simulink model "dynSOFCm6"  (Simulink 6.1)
settings: Solver=ode15s  StartTime=0.0  StopTime=1000  FixedStep=0.001  MinStep=1e-10  RelTol=1e-3
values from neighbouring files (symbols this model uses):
  A = 1e-4    (= 0.0001)    [dynSOFC_par.m]
  Aa = r3^2*(4-pi)    (= 0.000103867288916)    [dynSOFC_par.m]
  Ac = pi*(r2^2-r1^2)    (= 0.000122508290482)    [dynSOFC_par.m]
  At = pi*r0^2    (= 7.85398163397e-05)    [dynSOFC_par.m]
  C = 300e-6    (= 0.0003)    [dynSOFC_par.m]
  Cpc = 740    [dynSOFC_par.m]
  Cpt = 1217.7    [dynSOFC_par.m]
  D_a = 0.273*2*r3    (= 0.006006)    [dynSOFC_par.m]
  D_c = 2*(r2-r1)    (= 0.00532)    [dynSOFC_par.m]
  delta = 5.67e-8    (= 5.67e-08)    [dynSOFC_par.m]
  dVa = Aa*A/(2*pi*r3)    (= 1.50281749604e-07)    [dynSOFC_par.m]
  dVc = Ac*A/(2*pi*r3)    (= 1.77252727273e-07)    [dynSOFC_par.m]
  dVt = At*A/(2*pi*r3)    (= 1.13636363636e-07)    [dynSOFC_par.m]
  Ea = 1.1e5    (= 110000)    [dynSOFC_par.m]
  Ec = 1.2e5    (= 120000)    [dynSOFC_par.m]
  Ems1 = 0.4    [dynSOFC_par.m]
  Ems2 = 0.9    [dynSOFC_par.m]
  F = 96487    [dynSOFC_par.m]
  F21 = 0.69    [dynSOFC_par.m]
  K = 10    [dynSOFC_par.m]
  La = 0.1e-3    (= 0.0001)    [dynSOFC_par.m]
  Lc = 2.21e-3    (= 0.00221)    [dynSOFC_par.m]
  Le = 0.04e-3    (= 4e-05)    [dynSOFC_par.m]
  R = 8.314/101325    (= 8.20528003948e-05)    [dynSOFC_par.m]
  r0 = 5e-3    (= 0.005)    [dynSOFC_par.m]
  r1 = 6e-3    (= 0.006)    [dynSOFC_par.m]
  r2 = 8.66e-3    (= 0.00866)    [dynSOFC_par.m]
  r3 = 11e-3    (= 0.011)    [dynSOFC_par.m]
  Ro = 0.01    [dynSOFC_par.m]
  Rouc = 4592    [dynSOFC_par.m]
  Rout = 3900    [dynSOFC_par.m]
  x_ini = [    [dynSOFC_par.m]
libraries: simulink x25
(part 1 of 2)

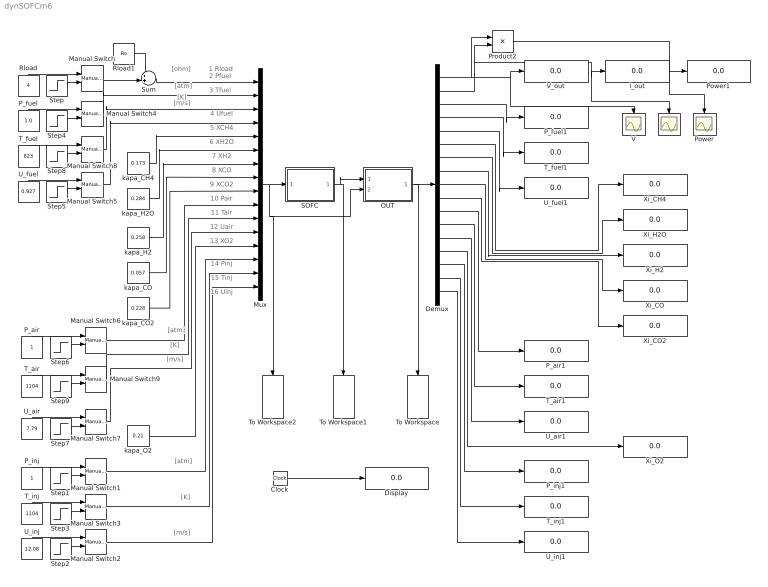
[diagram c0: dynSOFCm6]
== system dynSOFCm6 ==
  note: [ohm]
  note: [m/s]
  note: [atm]
  note: 1 Rload
  note: 3 Tfuel
  note: 5 XCH4
  note: [K]
  note: 6 XH2O
  note: 7 XH2
  note: 8 XCO
  note: 9 XCO2
  note: 4 Ufuel
  note: 2 Pfuel
  note: 10 Pair
  note: 11 Tair
  note: 12 Uair
  note: 13 XO2
  note: 14 Pinj
  note: 15 Tinj
  note: 16 Uinj
  note: [m/s]
  note: [atm]
  note: [K]
  note: [m/s]
  note: [atm]
  note: [K]
  Clock : Clock
  Demux : Demux  Outputs=17
  Display : Display
  I : Scope
  I_out : Display
  Manual Switch{,1..9} (10 alike) : simulink/Signal Routing/Manual Switch  sw=1  action=0
  Mux : Mux  Inputs=16
  OUT : Subsystem
  P_air : Constant  Orientation=up
  P_air1 : Display
  P_fuel : Constant  Orientation=up  Value=1.0
  P_fuel1 : Display
  P_inj : Constant  Orientation=up
  P_inj1 : Display
  Power : Scope
  Power1 : Display
  Product2 : Product
  Rload : Constant  Orientation=up  Value=4
  Rload1 : Constant  Value=Ro
  SOFC : Subsystem
  Step : Step  Time=100  Before=4  After=2
  Step1 : Step  Time=0.05  Before=0.03  After=0.03*0.5
  Step2 : Step  Time=0.05  Before=0.03  After=0.03*0.5
  Step3 : Step  Time=0.05  Before=0.03  After=0.03*0.5
  Step4 : Step  Time=100  Before=1  After=1.05
  Step5 : Step  Time=100  Before=0.927
  Step6 : Step  Time=100  Before=1  After=1.05
  Step7 : Step  Time=100  Before=7.79  After=8
  Step8 : Step  Time=100  Before=823  After=873
  Step9 : Step  Time=100  Before=1104  After=1154
  Sum : Sum  Inputs=++|
  T_air : Constant  Orientation=up  Value=1104
  T_air1 : Display
  T_fuel : Constant  Orientation=up  Value=823
  T_fuel1 : Display
  T_inj : Constant  Orientation=up  Value=1104
  T_inj1 : Display
  To Workspace : ToWorkspace  VariableName=y  SaveFormat=Array
  To Workspace1 : ToWorkspace  VariableName=x  SaveFormat=Array
  To Workspace2 : ToWorkspace  VariableName=u  SaveFormat=Array
  U_air : Constant  Orientation=up  Value=7.79
  U_air1 : Display
  U_fuel : Constant  Orientation=up  Value=0.927
  U_fuel1 : Display
  U_inj : Constant  Orientation=up  Value=12.08
  U_inj1 : Display
  V : Scope
  V_out : Display
  Xi_CH4 : Display
  Xi_CO : Display
  Xi_CO2 : Display
  Xi_H2 : Display
  Xi_H2O : Display
  Xi_O2 : Display
  kapa_CH4 : Constant  Value=0.173
  kapa_CO : Constant  Value=0.057
  kapa_CO2 : Constant  Value=0.228
  kapa_H2 : Constant  Value=0.258
  kapa_H2O : Constant  Value=0.284
  kapa_O2 : Constant  Value=0.21
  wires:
  Mux/1 -> SOFC/1(u), OUT/2(u), To Workspace2/1
  SOFC/1(x) -> OUT/1(x), To Workspace1/1
  OUT/1(y) -> Demux/1, To Workspace/1
  Demux/1 -> Product2/1, V_out/1, V/1
  Demux/2 -> Product2/2, I_out/1, I/1
  Rload/1 -> Manual Switch/1
  Step/1 -> Manual Switch/2
  Clock/1 -> Display/1
  Sum/1 -> Mux/1
  P_fuel/1 -> Manual Switch4/1
  Step4/1 -> Manual Switch4/2
  U_fuel/1 -> Manual Switch5/1
  Step5/1 -> Manual Switch5/2
  P_air/1 -> Manual Switch6/1
  Step6/1 -> Manual Switch6/2
  U_air/1 -> Manual Switch7/1
  Step7/1 -> Manual Switch7/2
  T_fuel/1 -> Manual Switch8/1
  Step8/1 -> Manual Switch8/2
  T_air/1 -> Manual Switch9/1
  Step9/1 -> Manual Switch9/2
  Manual Switch5/1 -> Mux/4
  Manual Switch4/1 -> Mux/2
  Manual Switch/1 -> Sum/2
  Rload1/1 -> Sum/1
  Manual Switch8/1 -> Mux/3
  P_inj/1 -> Manual Switch1/1
  U_inj/1 -> Manual Switch2/1
  Step2/1 -> Manual Switch2/2
  T_inj/1 -> Manual Switch3/1
  Step3/1 -> Manual Switch3/2
  kapa_CH4/1 -> Mux/5
  kapa_H2O/1 -> Mux/6
  kapa_H2/1 -> Mux/7
  kapa_CO/1 -> Mux/8
  kapa_CO2/1 -> Mux/9
  Manual Switch6/1 -> Mux/10
  Manual Switch9/1 -> Mux/11
  Manual Switch7/1 -> Mux/12
  kapa_O2/1 -> Mux/13
  Manual Switch1/1 -> Mux/14
  Manual Switch3/1 -> Mux/15
  Manual Switch2/1 -> Mux/16
  Product2/1 -> Power1/1, Power/1
  Demux/3 -> P_fuel1/1
  Demux/4 -> T_fuel1/1
  Demux/5 -> U_fuel1/1
  Demux/6 -> Xi_CH4/1
  Demux/7 -> Xi_H2O/1
  Demux/8 -> Xi_H2/1
  Demux/9 -> Xi_CO/1
  Demux/10 -> Xi_CO2/1
  Demux/11 -> P_air1/1
  Demux/12 -> T_air1/1
  Demux/13 -> U_air1/1
  Demux/14 -> Xi_O2/1
  Demux/15 -> P_inj1/1
  Demux/16 -> T_inj1/1
  Demux/17 -> U_inj1/1
  Step1/1 -> Manual Switch1/2

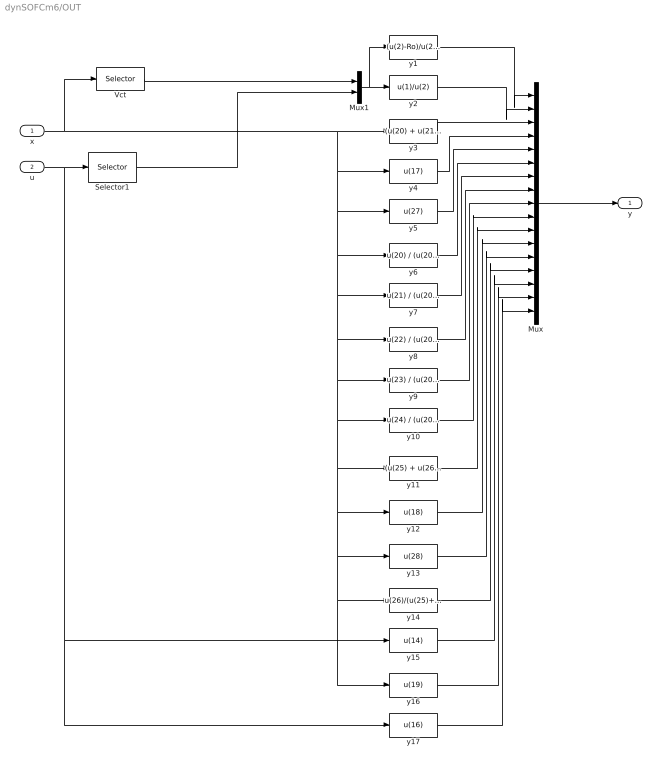
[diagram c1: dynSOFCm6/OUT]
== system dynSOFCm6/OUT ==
  x : Inport  Port=1  LatchInput=off
  u : Inport  Port=2  LatchInput=off
  Mux : Mux  Inputs=17
  Mux1 : Mux  Inputs=2
  Selector1 : Selector  Elements=[1]  InputPortWidth=16
  Vct : Selector  Elements=[1]  InputPortWidth=28
  y1 : Fcn  Expr=(u(2)-Ro)/u(2)*u(1)
  y10 : Fcn  Expr=u(24) / (u(20) + u(21) + u(22) + u(23) + u(24))
  y11 : Fcn  Expr=(u(25) + u(26)) * R * u(18) / dVc
  y12 : Fcn  Expr=u(18)
  y13 : Fcn  Expr=u(28)
  y14 : Fcn  Expr=u(26)/(u(25)+u(26))
  y15 : Fcn  Expr=u(14)
  y16 : Fcn  Expr=u(19)
  y17 : Fcn  Expr=u(16)
  y2 : Fcn  Expr=u(1)/u(2)
  y3 : Fcn  Expr=(u(20) + u(21) + u(22) + u(23) + u(24)) * R * u(17) /dVa
  y4 : Fcn  Expr=u(17)
  y5 : Fcn  Expr=u(27)
  y6 : Fcn  Expr=u(20) / (u(20) + u(21) + u(22) + u(23) + u(24))
  y7 : Fcn  Expr=u(21) / (u(20) + u(21) + u(22) + u(23) + u(24))
  y8 : Fcn  Expr=u(22) / (u(20) + u(21) + u(22) + u(23) + u(24))
  y9 : Fcn  Expr=u(23) / (u(20) + u(21) + u(22) + u(23) + u(24))
  y : Outport
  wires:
  x/1 -> Vct/1, y3/1, y4/1, y5/1, y6/1, y7/1, y8/1, y9/1, y10/1, y12/1, y13/1, y16/1, y14/1, y11/1
  u/1 -> Selector1/1, y15/1, y17/1
  y2/1 -> Mux/2
  Mux/1 -> y/1
  Selector1/1 -> Mux1/2
  Mux1/1 -> y2/1, y1/1
  y1/1 -> Mux/1
  Vct/1 -> Mux1/1
  y3/1 -> Mux/3
  y4/1 -> Mux/4
  y5/1 -> Mux/5
  y6/1 -> Mux/6
  y7/1 -> Mux/7
  y8/1 -> Mux/8
  y9/1 -> Mux/9
  y10/1 -> Mux/10
  y11/1 -> Mux/11
  y12/1 -> Mux/12
  y13/1 -> Mux/13
  y14/1 -> Mux/14
  y15/1 -> Mux/15
  y16/1 -> Mux/16
  y17/1 -> Mux/17

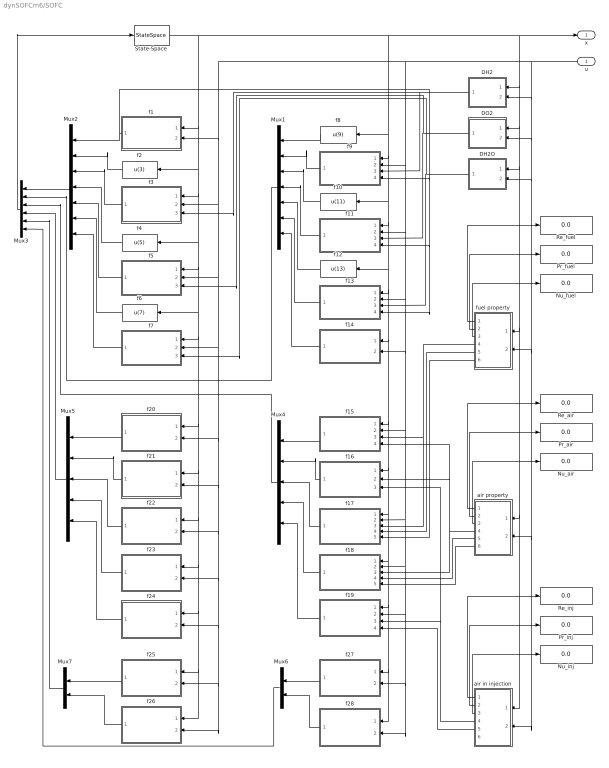
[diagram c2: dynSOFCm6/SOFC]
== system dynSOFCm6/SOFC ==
  u : Inport  Orientation=left  Port=1  LatchInput=off
  DH2 : Subsystem  Orientation=left
  DH2O : Subsystem  Orientation=left
  DO2 : Subsystem  Orientation=left
  Mux1 : Mux  Orientation=left  Inputs=7
  Mux2 : Mux  Orientation=left  Inputs=7
  Mux3 : Mux  Orientation=left  Inputs=6
  Mux4 : Mux  Orientation=left  Inputs=5
  Mux5 : Mux  Orientation=left  Inputs=5
  Mux6 : Mux  Orientation=left  Inputs=2
  Mux7 : Mux  Orientation=left  Inputs=2
  Nu_air : Display
  Nu_fuel : Display
  Nu_inj : Display
  Pr_air : Display
  Pr_fuel : Display
  Pr_inj : Display
  Re_air : Display
  Re_fuel : Display
  Re_inj : Display
  State-Space : StateSpace  A=zeros(28,28)  B=eye(28,28)  C=eye(28,28)  D=zeros(28,28)  X0=x_ini
  air in injection : Subsystem  Orientation=left
  air property : Subsystem  Orientation=left
  f1 : Subsystem  Orientation=left
  f10 : Fcn  Orientation=left  Expr=u(11)
  f11 : Subsystem  Orientation=left
  f12 : Fcn  Orientation=left  Expr=u(13)
  f13 : Subsystem  Orientation=left
  f14 : Subsystem  Orientation=left
  f15 : Subsystem  Orientation=left
  f16 : Subsystem  Orientation=left
  f17 : Subsystem  Orientation=left
  f18 : Subsystem  Orientation=left
  f19 : Subsystem  Orientation=left
  f2 : Fcn  Orientation=left  Expr=u(3)
  f20 : Subsystem  Orientation=left
  f21 : Subsystem  Orientation=left
  f22 : Subsystem  Orientation=left
  f23 : Subsystem  Orientation=left
  f24 : Subsystem  Orientation=left
  f25 : Subsystem  Orientation=left
  f26 : Subsystem  Orientation=left
  f27 : Subsystem  Orientation=left
  f28 : Subsystem  Orientation=left
  f3 : Subsystem  Orientation=left
  f4 : Fcn  Orientation=left  Expr=u(5)
  f5 : Subsystem  Orientation=left
  f6 : Fcn  Orientation=left  Expr=u(7)
  f7 : Subsystem  Orientation=left
  f8 : Fcn  Orientation=left  Expr=u(9)
  f9 : Subsystem  Orientation=left
  fuel property : Subsystem  Orientation=left
  x : Outport
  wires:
  State-Space/1 -> f1/1(x), f2/1, f3/1(x), f4/1, f5/1(x), f6/1, f7/1(x), f20/1(x), f21/1(x), f22/1(x), f23/1(x), f24/1(x), f26/1(x), f25/1(x), f8/1, f9/1(x), f10/1, f11/1(x), f13/1(x), f14/1(x), f15/1(x), f16/1(x), f17/1(x), f18/1(x), f19/1(x), f27/1(x), f28/1(x), f12/1, x/1, DH2/1(x), DO2/1(x), DH2O/1(x), fuel property/1(x), air property/1(x), air in injection/1(x)
  f3/1(dot x3) -> Mux2/3
  f2/1 -> Mux2/2
  f1/1(dot x1) -> Mux2/1, f9/4(dotx1), f11/4(dot x1), f13/4(dot x1)
  f4/1 -> Mux2/4
  f5/1(dot x5) -> Mux2/5
  f6/1 -> Mux2/6
  f7/1(dot x7) -> Mux2/7
  f8/1 -> Mux1/1
  f9/1(dot x9) -> Mux1/2
  f10/1 -> Mux1/3
  f11/1(dot x11) -> Mux1/4
  f12/1 -> Mux1/5
  f13/1(dot x13) -> Mux1/6
  f14/1(dot x14) -> Mux1/7
  Mux2/1 -> Mux3/1
  Mux3/1 -> State-Space/1
  u/1 -> f1/2(u), f3/2(u), f5/2(u), f7/2(u), f20/2(u), f21/2(u), f22/2(u), f23/2(u), f24/2(u), f26/2(u), f25/2(u), f9/2(u), f13/2(u), f14/2(u), f15/2(u), f17/2(u), f18/2(u), f19/2(u), f27/2(u), f28/2(u), f11/2(u), DH2/2(u), DO2/2(u), DH2O/2(u), fuel property/2(u), air property/2(u), air in injection/2(u)
  DH2/1(DH2) -> f3/3(DH2), f9/3(DH2)
  DO2/1(DO2) -> f5/3(DO2), f11/3(DO2)
  DH2O/1(DH2O) -> f7/3(DH2O), f13/3(DH2O)
  Mux1/1 -> Mux3/2
  fuel property/4(h_fuel) -> f15/3(ha), f17/3(ha)
  air in injection/4(h_inj) -> f16/3(h_t), f19/3(ht)
  fuel property/5(N*Cv) -> f17/4(fuel (Ni*Cvi))
  fuel property/6(d(N*Cv)/dt) -> f17/5(fuel d(Ni*Cvi))
  air in injection/5(N*Cv) -> f19/4(inj (Ni*Cvi))
  air property/5(N*Cv) -> f18/4(air (Ni*Cvi))
  air property/6(d(N*Cv)) -> f18/5(air d(Ni*Cvi))
  f15/1(dot x15) -> Mux4/1
  f16/1(dot x16) -> Mux4/2
  f17/1(dot x17) -> Mux4/3
  f18/1(dot x18) -> Mux4/4
  f19/1(dot x19) -> Mux4/5
  f20/1(dot x20) -> Mux5/1
  f21/1(dot x21) -> Mux5/2
  f22/1(dot x22) -> Mux5/3
  f23/1(dot x23) -> Mux5/4
  f24/1(dot x24) -> Mux5/5
  f27/1(dot x27) -> Mux6/1
  f28/1(dot x28) -> Mux6/2
  Mux4/1 -> Mux3/3
  Mux5/1 -> Mux3/4
  Mux6/1 -> Mux3/6
  air property/1(Re_air) -> Re_air/1
  air property/2(Pr_air) -> Pr_air/1
  air property/3(Nu_air) -> Nu_air/1
  fuel property/1(Re_fuel) -> Re_fuel/1
  fuel property/2(Pr_fuel) -> Pr_fuel/1
  fuel property/3(Nu_fuel) -> Nu_fuel/1
  air in injection/1(Re_inj) -> Re_inj/1
  air in injection/2(Pr_inj) -> Pr_inj/1
  air in injection/3(Nu_inj) -> Nu_inj/1
  f25/1(dot x25) -> Mux7/1
  f26/1(dot x26) -> Mux7/2
  Mux7/1 -> Mux3/5
  air property/4(h_air) -> f18/3(hc), f16/2(hc), f15/4(hc)

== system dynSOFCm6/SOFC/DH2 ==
  x : Inport  Port=1  LatchInput=off
  u : Inport  Port=2  LatchInput=off
  D : Fcn  Expr=4.17e-5*u(1)^1.75/u(2)/101325
  Mux1 : Mux  Inputs=2
  Pfuel : Selector  Elements=[2]  InputPortWidth=16
  Tcell : Selector  Elements=[15]  InputPortWidth=28
  DH2 : Outport
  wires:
  Pfuel/1 -> Mux1/2
  u/1 -> Pfuel/1
  x/1 -> Tcell/1
  Tcell/1 -> Mux1/1
  Mux1/1 -> D/1
  D/1 -> DH2/1

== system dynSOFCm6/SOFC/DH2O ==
  x : Inport  Port=1  LatchInput=off
  u : Inport  Port=2  LatchInput=off
  D : Fcn  Expr=4.17e-5*u(1)^1.75/u(2)/101325
  Mux1 : Mux  Inputs=2
  Pfuel : Selector  Elements=[2]  InputPortWidth=16
  Tcell : Selector  Elements=[15]  InputPortWidth=28
  DH2O : Outport
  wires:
  D/1 -> DH2O/1
  Mux1/1 -> D/1
  Tcell/1 -> Mux1/1
  x/1 -> Tcell/1
  u/1 -> Pfuel/1
  Pfuel/1 -> Mux1/2

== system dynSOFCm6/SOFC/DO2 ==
  x : Inport  Port=1  LatchInput=off
  u : Inport  Port=2  LatchInput=off
  D : Fcn  Expr=9.82e-6*u(1)^1.75/u(2)/101325
  Mux1 : Mux  Inputs=2
  Pair : Selector  Elements=[10]  InputPortWidth=16
  Tcell : Selector  Elements=[15]  InputPortWidth=28
  DO2 : Outport
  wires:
  D/1 -> DO2/1
  Mux1/1 -> D/1
  Tcell/1 -> Mux1/1
  x/1 -> Tcell/1
  u/1 -> Pair/1
  Pair/1 -> Mux1/2

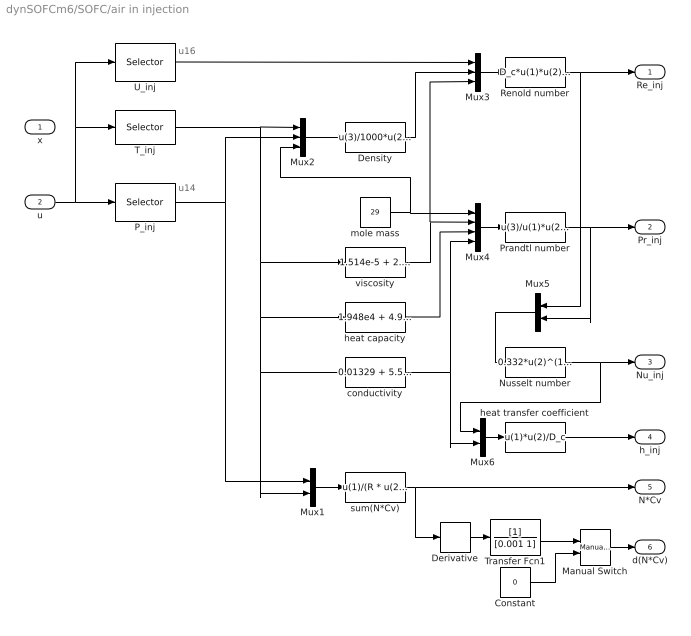
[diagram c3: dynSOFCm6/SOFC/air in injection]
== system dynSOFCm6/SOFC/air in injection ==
  note: u16
  note: u14
  x : Inport  Port=1  LatchInput=off
  u : Inport  Port=2  LatchInput=off
  Constant : Constant  Value=0
  Density : Fcn  Expr=u(3)/1000*u(2)/R/u(1)
  Derivative : Derivative
  Manual Switch : simulink/Signal Routing/Manual Switch  sw=1  action=0
  Mux1 : Mux  Inputs=2
  Mux2 : Mux  Inputs=3
  Mux3 : Mux  Inputs=3
  Mux4 : Mux
  Mux5 : Mux  Orientation=left  Inputs=2
  Mux6 : Mux  Inputs=2
  Nusselt number : Fcn  Expr=0.332*u(2)^(1/3)*u(1)^(1/2)
  P_inj : Selector  Elements=[14]  InputPortWidth=16
  Prandtl number : Fcn  Expr=u(3)/u(1)*u(2)/u(4)
  Renold number : Fcn  Expr=D_c*u(1)*u(2)/u(3)
  T_inj : Selector  Elements=[15]  InputPortWidth=16
  Transfer Fcn1 : TransferFcn  Denominator=[0.001 1]
  U_inj : Selector  Elements=[16]  InputPortWidth=16
  conductivity : Fcn  Expr=0.01329 + 5.539e-5*u(1)
  heat capacity : Fcn  Expr=1.948e4 + 4.936*u(1)
  heat transfer coefficient : Fcn  Expr=u(1)*u(2)/D_c
  mole mass : Constant  Value=29
  sum(N*Cv) : Fcn  Expr=u(1)/(R * u(2)) * dVt * (1.948e4 + 4.936 * u(2))/1000
  viscosity : Fcn  Expr=1.514e-5 + 2.793e-8*u(1)
  Re_inj : Outport
  Pr_inj : Outport  Port=2
  Nu_inj : Outport  Port=3
  h_inj : Outport  Port=4
  N*Cv : Outport  Port=5
  d(N*Cv) : Outport  Port=6
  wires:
  u/1 -> P_inj/1, U_inj/1, T_inj/1
  Nusselt number/1 -> Nu_inj/1, Mux6/1
  Mux5/1 -> Nusselt number/1
  Prandtl number/1 -> Mux5/2, Pr_inj/1
  conductivity/1 -> Mux4/4, Mux6/2
  heat capacity/1 -> Mux4/3
  Mux4/1 -> Prandtl number/1
  viscosity/1 -> Mux4/2, Mux3/3
  mole mass/1 -> Mux4/1, Mux2/3
  P_inj/1 -> Mux2/2, Mux1/1
  Renold number/1 -> Mux5/1, Re_inj/1
  Mux3/1 -> Renold number/1
  Density/1 -> Mux3/2
  Mux2/1 -> Density/1
  U_inj/1 -> Mux3/1
  T_inj/1 -> Mux2/1, heat capacity/1, conductivity/1, Mux1/2, viscosity/1
  Mux6/1 -> heat transfer coefficient/1
  heat transfer coefficient/1 -> h_inj/1
  Mux1/1 -> sum(N*Cv)/1
  sum(N*Cv)/1 -> N*Cv/1, Derivative/1
  Constant/1 -> Manual Switch/2
  Manual Switch/1 -> d(N*Cv)/1
  Derivative/1 -> Transfer Fcn1/1
  Transfer Fcn1/1 -> Manual Switch/1

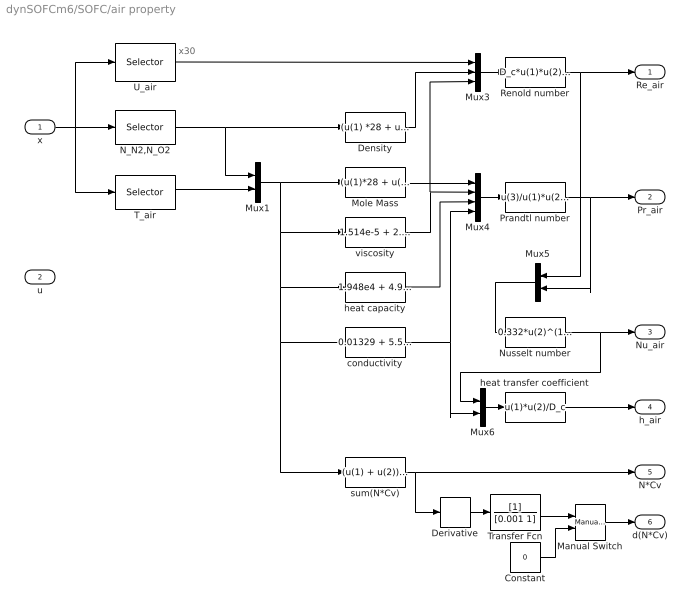
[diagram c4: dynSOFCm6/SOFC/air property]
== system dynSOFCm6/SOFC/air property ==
  note: x30
  x : Inport  Port=1  LatchInput=off
  u : Inport  Port=2  LatchInput=off
  Constant : Constant  Value=0
  Density : Fcn  Expr=(u(1) *28 + u(2)*32) / dVc /1000
  Derivative : Derivative
  Manual Switch : simulink/Signal Routing/Manual Switch  sw=1  action=0
  Mole Mass : Fcn  Expr=(u(1)*28 + u(2)*32)/(u(1) +u(2) )
  Mux1 : Mux  Inputs=2
  Mux3 : Mux  Inputs=3
  Mux4 : Mux
  Mux5 : Mux  Orientation=left  Inputs=2
  Mux6 : Mux  Inputs=2
  N_N2,N_O2 : Selector  Elements=[25 26]  InputPortWidth=28
  Nusselt number : Fcn  Expr=0.332*u(2)^(1/3)*u(1)^(1/2)
  Prandtl number : Fcn  Expr=u(3)/u(1)*u(2)/u(4)
  Renold number : Fcn  Expr=D_c*u(1)*u(2)/u(3)
  T_air : Selector  Elements=[18]  InputPortWidth=28
  Transfer Fcn : TransferFcn  Denominator=[0.001 1]
  U_air : Selector  Elements=[28]  InputPortWidth=28
  conductivity : Fcn  Expr=0.01329 + 5.539e-5*u(3)
  heat capacity : Fcn  Expr=1.948e4 + 4.936*u(3)
  heat transfer coefficient : Fcn  Expr=u(1)*u(2)/D_c
  sum(N*Cv) : Fcn  Expr="(u(1) + u(2)) *  (1.948e4 + 4.936*u(3))/1000"
  viscosity : Fcn  Expr=1.514e-5 + 2.793e-8*u(3)
  Re_air : Outport
  Pr_air : Outport  Port=2
  Nu_air : Outport  Port=3
  h_air : Outport  Port=4
  N*Cv : Outport  Port=5
  d(N*Cv) : Outport  Port=6
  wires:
  heat transfer coefficient/1 -> h_air/1
  Mux6/1 -> heat transfer coefficient/1
  N_N2,N_O2/1 -> Mux1/1, Density/1
  U_air/1 -> Mux3/1
  Density/1 -> Mux3/2
  Mux3/1 -> Renold number/1
  Renold number/1 -> Re_air/1, Mux5/1
  x/1 -> U_air/1, N_N2,N_O2/1, T_air/1
  Mole Mass/1 -> Mux4/1
  viscosity/1 -> Mux3/3, Mux4/2
  Mux4/1 -> Prandtl number/1
  heat capacity/1 -> Mux4/3
  conductivity/1 -> Mux6/2, Mux4/4
  Prandtl number/1 -> Pr_air/1, Mux5/2
  Mux5/1 -> Nusselt number/1
  Nusselt number/1 -> Mux6/1, Nu_air/1
  sum(N*Cv)/1 -> N*Cv/1, Derivative/1
  Constant/1 -> Manual Switch/2
  Manual Switch/1 -> d(N*Cv)/1
  Mux1/1 -> Mole Mass/1, viscosity/1, heat capacity/1, conductivity/1, sum(N*Cv)/1
  T_air/1 -> Mux1/2
  Derivative/1 -> Transfer Fcn/1
  Transfer Fcn/1 -> Manual Switch/1

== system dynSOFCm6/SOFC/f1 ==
  x : Inport  Port=1  LatchInput=off
  u : Inport  Port=2  LatchInput=off
  Divide : Product  Inputs=*/  OutScaling=2^-10
  E : Subsystem
  Fcn : Fcn  Expr=1/u(1)
  Gain1 : Gain  Gain=1/C
  Product : Product
  Rct*C : Fcn  Expr=2.94e-5*exp(10350/u(1)) *Le/A*C
  Selector : Selector  Elements=[1]  InputPortWidth=28
  Selector1 : Selector  Elements=[1]  InputPortWidth=16
  Selector2 : Selector  Elements=[15]  InputPortWidth=28
  Sum : Sum  Inputs=|+-
  Sum1 : Sum  Inputs=|+-
  dot x1 : Outport
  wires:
  E/1(E) -> Sum/1
  x/1 -> Selector/1, Selector2/1, E/1(x)
  Selector/1 -> Sum/2, Product/1
  u/1 -> Selector1/1, E/2(u)
  Selector1/1 -> Fcn/1
  Fcn/1 -> Product/2
  Product/1 -> Gain1/1
  Gain1/1 -> Sum1/2
  Sum1/1 -> dot x1/1
  Sum/1 -> Divide/1
  Divide/1 -> Sum1/1
  Selector2/1 -> Rct*C/1
  Rct*C/1 -> Divide/2

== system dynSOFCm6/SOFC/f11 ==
  note: 11
  note: 1-4
  note: 5-6
  note: 7-10
  note: 12
  note: x18,26
  note: u1
  note: x1,10,11,14
  note: x15
  x : Inport  Port=1  LatchInput=off
  u : Inport  Port=2  LatchInput=off
  DO2 : Inport  Port=3  LatchInput=off
  dot x1 : Inport  Port=4  LatchInput=off
  Ex11 : Fcn  Expr=-u(7)*u(2) - u(8)*u(3) - R*u(12)/A/(4*F)*u(10)*u(1)/u(5) + u(7)*u(6) - R*u(12)/A*4/Lc/(4*F)*(u(11)/u(5) - u(1)/(u(5)^2)*(K*u(5)-u(4)))
  Mux : Mux
  Mux1 : Mux  Inputs=5
  Mux2 : Mux  Inputs=2
  Rload+Ro : Selector  Elements=[1]  InputPortWidth=16
  "Tair, NO2" : Selector  Elements=[18 26 ]  InputPortWidth=28
  Tcell : Selector  Elements=[15]  InputPortWidth=28
  a1 : Fcn  Expr=24*u(1)^2/(Lc^4)
  a2 : Fcn  Expr=12*u(1)/(Lc^2)
  a3 : Fcn  Expr=24*u(1)^2/(Lc^3)
  a4 : Fcn  Expr=24*u(1)/(Lc^3)
  pbO2 : Fcn  Expr=u(2)*u(1)*R/dVc
  ptO2 : Selector  Elements=[1 10 11 14]  InputPortWidth=28
  dot x11 : Outport
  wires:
  dot x1/1 -> Mux1/4
  x/1 -> ptO2/1, Tcell/1, "Tair, NO2"/1
  DO2/1 -> a1/1, a2/1, a4/1, a3/1
  a1/1 -> Mux/1
  a2/1 -> Mux/2
  a3/1 -> Mux/3
  a4/1 -> Mux/4
  ptO2/1 -> Mux1/1
  Mux/1 -> Mux1/3
  Mux1/1 -> Ex11/1
  Ex11/1 -> dot x11/1
  Tcell/1 -> Mux1/5
  "Tair, NO2"/1 -> pbO2/1
  Rload+Ro/1 -> Mux2/1
  pbO2/1 -> Mux2/2
  Mux2/1 -> Mux1/2
  u/1 -> Rload+Ro/1

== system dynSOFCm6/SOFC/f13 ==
  note: 11
  note: 1-4
  note: 5-6
  note: 7-10
  note: 12
  note: u1
  note: x17,21
  note: x1,12,13,14
  note: x15
  x : Inport  Port=1  LatchInput=off
  u : Inport  Port=2  LatchInput=off
  DH2O : Inport  Port=3  LatchInput=off
  dot x1 : Inport  Port=4  LatchInput=off
  Ex13 : Fcn  Expr=-u(7)*u(2) - u(8)*u(3) + R*u(12)/A/(2*F)*u(10)*u(1)/u(5) + u(7)*u(6) + R*u(12)/A*4/La/(2*F)*(u(11)/u(5) - u(1)/(u(5)^2)*(K*u(5)-u(4)))
  Mux : Mux
  Mux1 : Mux  Inputs=5
  Mux3 : Mux  Inputs=2
  Rload+Ro1 : Selector  Elements=[1]  InputPortWidth=16
  Tcell : Selector  Elements=[15]  InputPortWidth=28
  "Tfuel, NH2O" : Selector  Elements=[17 21 ]  InputPortWidth=28
  a1 : Fcn  Expr=24*u(1)^2/(La^4)
  a2 : Fcn  Expr=12*u(1)/(La^2)
  a3 : Fcn  Expr=24*u(1)^2/(La^3)
  a4 : Fcn  Expr=24*u(1)/(La^3)
  pbH2O : Fcn  Expr=u(2)*u(1)*R/dVa
  ptH2O : Selector  Elements=[1 12 13 14]  InputPortWidth=28
  dot x13 : Outport
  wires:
  dot x1/1 -> Mux1/4
  x/1 -> ptH2O/1, Tcell/1, "Tfuel, NH2O"/1
  DH2O/1 -> a1/1, a2/1, a4/1, a3/1
  a1/1 -> Mux/1
  a2/1 -> Mux/2
  a3/1 -> Mux/3
  a4/1 -> Mux/4
  ptH2O/1 -> Mux1/1
  Mux/1 -> Mux1/3
  Mux1/1 -> Ex13/1
  Ex13/1 -> dot x13/1
  Tcell/1 -> Mux1/5
  "Tfuel, NH2O"/1 -> pbH2O/1
  Rload+Ro1/1 -> Mux3/1
  pbH2O/1 -> Mux3/2
  Mux3/1 -> Mux1/2
  u/1 -> Rload+Ro1/1

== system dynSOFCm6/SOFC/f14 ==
  x : Inport  Port=1  LatchInput=off
  u : Inport  Port=2  LatchInput=off
  Gain : Gain  Gain=K
  Gain1 : Gain  Gain=K^2
  Selector : Selector  Elements=[14]  InputPortWidth=28
  Selector1 : Selector  Elements=[1]  InputPortWidth=16
  Sum : Sum  Inputs=|-+
  dot x14 : Outport
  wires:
  Gain1/1 -> Sum/2
  Gain/1 -> Sum/1
  Selector1/1 -> Gain1/1
  Selector/1 -> Gain/1
  u/1 -> Selector1/1
  x/1 -> Selector/1
  Sum/1 -> dot x14/1

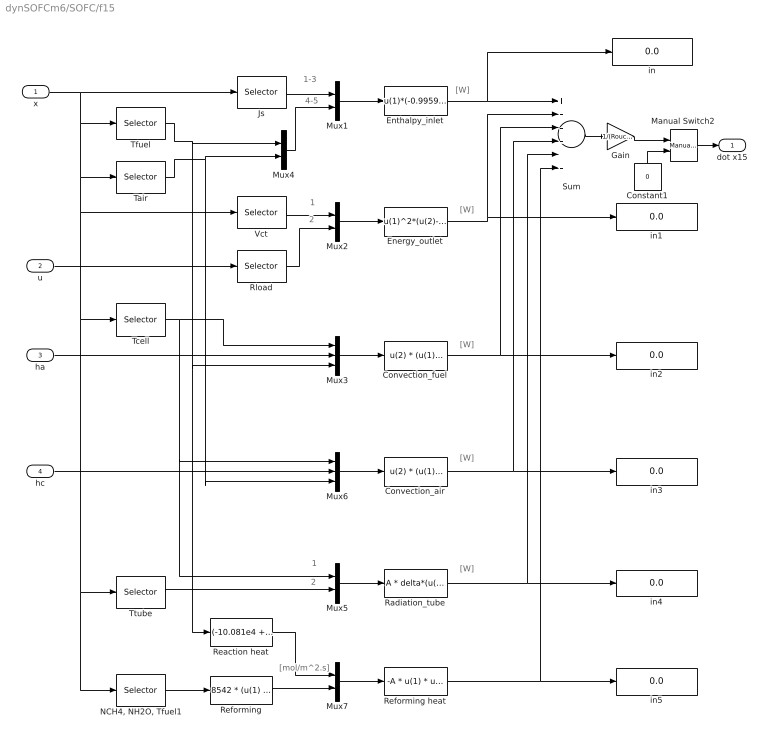
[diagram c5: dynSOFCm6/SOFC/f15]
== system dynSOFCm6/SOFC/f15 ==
  note: 1-3
  note: 4-5
  note: 1
  note: 2
  note: 1
  note: 2
  note: [W]
  note: [W]
  note: [W]
  note: [W]
  note: [W]
  note: [mol/m^2.s]
  x : Inport  Port=1  LatchInput=off
  u : Inport  Port=2  LatchInput=off
  ha : Inport  Port=3  LatchInput=off
  hc : Inport  Port=4  LatchInput=off
  Constant1 : Constant  Orientation=up  Value=0
  Convection_air : Fcn  Expr=u(2) * (u(1) - u(3)) * A *r2/r3
  Convection_fuel : Fcn  Expr=u(2) * (u(1) - u(3)) * A
  Energy_outlet : Fcn  Expr=u(1)^2*(u(2)-Ro)/(u(2)^2)
  Enthalpy_inlet : Fcn  Expr="u(1)*(-0.9959e4+30.73*u(4)) + u(2)*(-1.2290e4+35.12*u(5))  + u(3)*(-25.790e4+42.47*u(4))"
  Gain : Gain  Gain=1/(Rouc*Cpc*(r3-r2)*A)
  Js : Selector  Elements=[2 4 6]  InputPortWidth=28
  Manual Switch2 : simulink/Signal Routing/Manual Switch  sw=1  action=0
  Mux{1..2,4..5,7} (5 alike) : Mux  Inputs=2
  Mux3 : Mux  Inputs=3
  Mux6 : Mux  Inputs=3
  "NCH4, NH2O, Tfuel1" : Selector  Elements=[20 21 17]  InputPortWidth=28
  Radiation_tube : Fcn  Expr=A * delta*(u(1)^4-u(2)^4)/((1-Ems2)/Ems2 + 1/F21 + (1-Ems1)/Ems1*(r2/r1)^2)
  Reaction heat : Fcn  Expr="(-10.081e4 + 62.12 * u(1)) +  (-25.79e4 + 42.47 * u(1)) - 3* (-0.9959e4 + 30.73*u(1))  -  (-12.150e4 + 31.81* u(1))"
  Reforming : Fcn  Expr=8542 * (u(1) * R * u(3) / dVa )^(0.85) * (u(2) * R * u(3) / dVa )^(-0.35) * exp( -95e3 /(8.314*u(3)) )
  Reforming heat : Fcn  Expr=-A * u(1) * u(2)
  Rload : Selector  Elements=[1]  InputPortWidth=16
  Sum : Sum  Inputs=+-----
  Tair : Selector  Elements=[18]  InputPortWidth=28
  Tcell : Selector  Elements=[15]  InputPortWidth=28
  Tfuel : Selector  Elements=[17]  InputPortWidth=28
  Ttube : Selector  Elements=[16]  InputPortWidth=28
  Vct : Selector  Elements=[1]  InputPortWidth=28
  in{,1..5} (6 alike) : Display
  dot x15 : Outport
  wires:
  x/1 -> Js/1, Tfuel/1, Vct/1, Tcell/1, Ttube/1, "NCH4, NH2O, Tfuel1"/1, Tair/1
  Js/1 -> Mux1/1
  Mux1/1 -> Enthalpy_inlet/1
  Mux4/1 -> Mux1/2
  Vct/1 -> Mux2/1
  Rload/1 -> Mux2/2
  Mux2/1 -> Energy_outlet/1
  Mux3/1 -> Convection_fuel/1
  Mux5/1 -> Radiation_tube/1
  Tcell/1 -> Mux3/1, Mux5/1, Mux6/1
  u/1 -> Rload/1
  Enthalpy_inlet/1 -> Sum/1, in/1
  Energy_outlet/1 -> Sum/2, in1/1
  Convection_fuel/1 -> Sum/3, in2/1
  Convection_air/1 -> Sum/4, in3/1
  Radiation_tube/1 -> Sum/5, in4/1
  Mux6/1 -> Convection_air/1
  Tfuel/1 -> Mux4/1, Mux3/3, Reaction heat/1
  ha/1 -> Mux3/2
  hc/1 -> Mux6/2
  Tair/1 -> Mux6/3, Mux4/2
  Ttube/1 -> Mux5/2
  "NCH4, NH2O, Tfuel1"/1 -> Reforming/1
  Mux7/1 -> Reforming heat/1
  Reforming/1 -> Mux7/2
  Reaction heat/1 -> Mux7/1
  Reforming heat/1 -> Sum/6, in5/1
  Sum/1 -> Gain/1
  Gain/1 -> Manual Switch2/1
  Constant1/1 -> Manual Switch2/2
  Manual Switch2/1 -> dot x15/1

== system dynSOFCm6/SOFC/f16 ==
  note: [W]
  note: [W]
  note: [W]
  x : Inport  Port=1  LatchInput=off
  hc : Inport  Port=2  LatchInput=off
  h_t : Inport  Port=3  LatchInput=off
  Constant1 : Constant  Orientation=up  Value=0
  Convection_air : Fcn  Expr=u(3) * (u(2) - u(1)) * A * r1 / r3
  Convection_inj : Fcn  Expr=u(3) * (u(1) - u(2)) * A * r0 / r3
  Gain : Gain  Gain=1/(Rout*Cpt*(r1-r0)*A*r1/r3)
  Manual Switch2 : simulink/Signal Routing/Manual Switch  sw=1  action=0
  Mux3 : Mux  Inputs=3
  Mux5 : Mux  Inputs=2
  Mux6 : Mux  Inputs=3
  Radiation_tube : Fcn  Expr=A * delta*(u(1)^4-u(2)^4)/((1-Ems2)/Ems2 + 1/F21 + (1-Ems1)/Ems1*(r2/r1)^2)
  Sum : Sum  Inputs=+--
  Tair : Selector  Elements=[18]  InputPortWidth=28
  Tcell : Selector  Elements=[15]  InputPortWidth=28
  Tinj : Selector  Elements=[19]  InputPortWidth=28
  Ttube : Selector  Elements=[16]  InputPortWidth=28
  in1 : Display
  in2 : Display
  in3 : Display
  dot x16 : Outport
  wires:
  Mux6/1 -> Convection_inj/1
  Radiation_tube/1 -> in1/1, Sum/1
  Convection_inj/1 -> in3/1, Sum/3
  Convection_air/1 -> in2/1, Sum/2
  Mux5/1 -> Radiation_tube/1
  Mux3/1 -> Convection_air/1
  x/1 -> Tcell/1, Tair/1, Tinj/1, Ttube/1
  Tair/1 -> Mux3/1
  Tcell/1 -> Mux5/1
  Ttube/1 -> Mux5/2, Mux3/2, Mux6/1
  hc/1 -> Mux3/3
  Tinj/1 -> Mux6/2
  h_t/1 -> Mux6/3
  Sum/1 -> Gain/1
  Constant1/1 -> Manual Switch2/2
  Gain/1 -> Manual Switch2/1
  Manual Switch2/1 -> dot x16/1

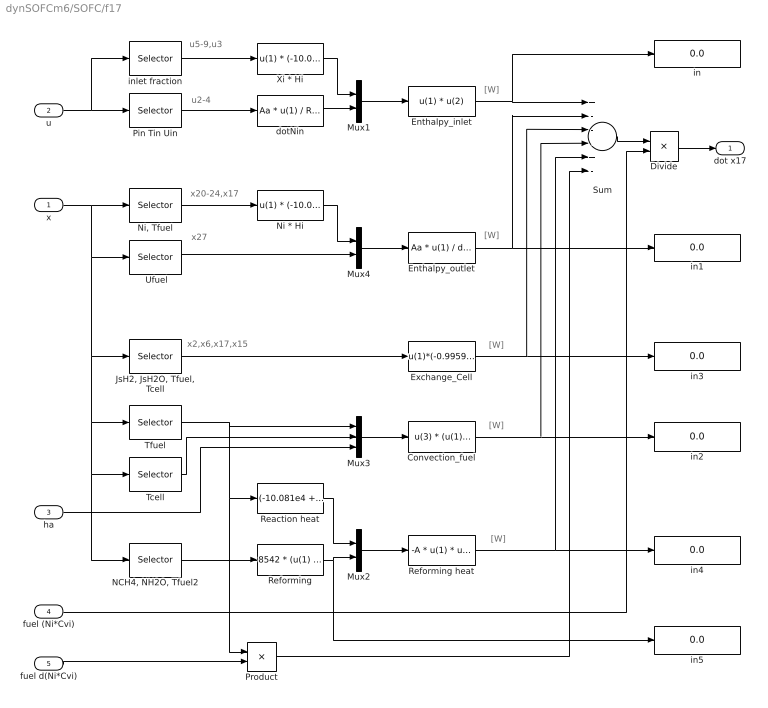
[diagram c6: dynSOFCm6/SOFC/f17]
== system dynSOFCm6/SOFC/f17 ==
  note: [W]
  note: [W]
  note: [W]
  note: u5-9,u3
  note: u2-4
  note: x20-24,x17
  note: [W]
  note: x27
  note: x2,x6,x17,x15
  note: [W]
  x : Inport  Port=1  LatchInput=off
  u : Inport  Port=2  LatchInput=off
  ha : Inport  Port=3  LatchInput=off
  fuel (Ni*Cvi) : Inport  Port=4  LatchInput=off
  fuel d(Ni*Cvi) : Inport  Port=5  LatchInput=off
  " Ufuel" : Selector  Elements=[27]  InputPortWidth=28
  Convection_fuel : Fcn  Expr=u(3) * (u(1) - u(2)) * A
  Divide : Product  Inputs=*/  OutScaling=2^-10
  Enthalpy_inlet : Fcn  Expr=u(1) * u(2)
  Enthalpy_outlet : Fcn  Expr=Aa * u(1) / dVa * u(2)
  Exchange_Cell : Fcn  Expr="u(1)*(-0.9959e4+30.73*u(3))   + u(2)*(-25.790e4+42.47*u(4))"
  "JsH2, JsH2O, Tfuel, Tcell" : Selector  Elements=[2 6 17 15]  InputPortWidth=28
  Mux1 : Mux  Inputs=2
  Mux2 : Mux  Inputs=2
  Mux3 : Mux  Inputs=3
  Mux4 : Mux  Inputs=2
  "NCH4, NH2O, Tfuel2" : Selector  Elements=[20 21 17]  InputPortWidth=28
  Ni * Hi : Fcn  Expr=u(1) * (-10.081e4 + 62.12 * u(6)) + u(2) * (-25.79e4 + 42.47 * u(6)) + u(3) * (-0.9959e4 + 30.73*u(6)) + u(4) * (-12.150e4 + 31.81* u(6)) + u(5) * (-41.700e4 + 50.89 * u(6))
  "Ni, Tfuel" : Selector  Elements=[20 21 22 23 24 17]  InputPortWidth=28
  Pin Tin Uin : Selector  Elements=[2 3 4]  InputPortWidth=16
  Product : Product
  Reaction heat : Fcn  Expr="(-10.081e4 + 62.12 * u(1)) +  (-25.79e4 + 42.47 * u(1)) - 3* (-0.9959e4 + 30.73*u(1))  -  (-12.150e4 + 31.81* u(1))"
  Reforming : Fcn  Expr=8542 * (u(1) * R * u(3) / dVa )^(0.85) * (u(2) * R * u(3) / dVa )^(-0.35) * exp( -95e3 /(8.314*u(3)) )
  Reforming heat : Fcn  Expr=-A * u(1) * u(2)
  Sum : Sum  Inputs=+---+-
  Tcell : Selector  Elements=[15]  InputPortWidth=28
  Tfuel : Selector  Elements=[17]  InputPortWidth=28
  Xi * Hi : Fcn  Expr=u(1) * (-10.081e4 + 62.12 * u(6)) + u(2) * (-25.79e4 + 42.47 * u(6)) + u(3) * (-0.9959e4 + 30.73*u(6)) + u(4) * (-12.150e4 + 31.81* u(6)) + u(5) * (-41.700e4 + 50.89 * u(6))
  dotNin : Fcn  Expr=Aa * u(1) / R / u(2) * u(3)
  in{,1..5} (6 alike) : Display
  inlet fraction : Selector  Elements=[5 6 7 8 9 3]  InputPortWidth=16
  dot x17 : Outport
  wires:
  Sum/1 -> Divide/1
  Convection_fuel/1 -> in2/1, Sum/4
  Enthalpy_outlet/1 -> in1/1, Sum/2
  Enthalpy_inlet/1 -> Sum/1, in/1
  u/1 -> inlet fraction/1, Pin Tin Uin/1
  Tcell/1 -> Mux3/2
  Mux3/1 -> Convection_fuel/1
  Mux1/1 -> Enthalpy_inlet/1
  inlet fraction/1 -> Xi * Hi/1
  x/1 -> "Ni, Tfuel"/1, " Ufuel"/1, "JsH2, JsH2O, Tfuel, Tcell"/1, Tfuel/1, Tcell/1, "NCH4, NH2O, Tfuel2"/1
  Pin Tin Uin/1 -> dotNin/1
  Xi * Hi/1 -> Mux1/1
  dotNin/1 -> Mux1/2
  "Ni, Tfuel"/1 -> Ni * Hi/1
  Ni * Hi/1 -> Mux4/1
  Mux4/1 -> Enthalpy_outlet/1
  "JsH2, JsH2O, Tfuel, Tcell"/1 -> Exchange_Cell/1
  Tfuel/1 -> Mux3/1, Reaction heat/1, Product/1
  ha/1 -> Mux3/3
  fuel (Ni*Cvi)/1 -> Divide/2
  "NCH4, NH2O, Tfuel2"/1 -> Reforming/1
  Mux2/1 -> Reforming heat/1
  Reaction heat/1 -> Mux2/1
  Reforming/1 -> Mux2/2, in5/1
  " Ufuel"/1 -> Mux4/2
  Exchange_Cell/1 -> in3/1, Sum/3
  Reforming heat/1 -> in4/1, Sum/5
  fuel d(Ni*Cvi)/1 -> Product/2
  Product/1 -> Sum/6
  Divide/1 -> dot x17/1

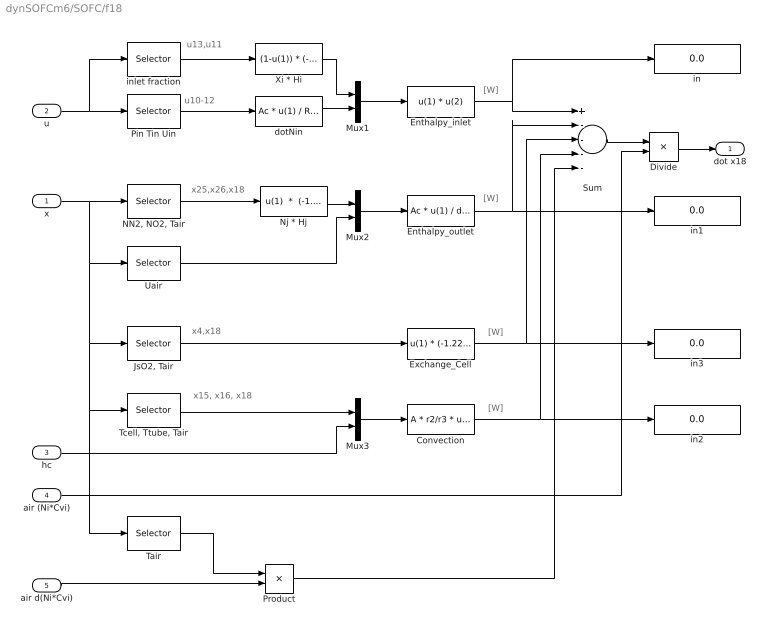
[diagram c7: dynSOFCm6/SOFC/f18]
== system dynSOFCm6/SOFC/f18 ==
  note: x4,x18
  note: [W]
  note: x25,x26,x18
  note: u10-12
  note: u13,u11
  note: [W]
  note: [W]
  note: [W]
  note: x15, x16, x18
  x : Inport  Port=1  LatchInput=off
  u : Inport  Port=2  LatchInput=off
  hc : Inport  Port=3  LatchInput=off
  air (Ni*Cvi) : Inport  Port=4  LatchInput=off
  air d(Ni*Cvi) : Inport  Port=5  LatchInput=off
  Convection : Fcn  Expr=A * r2/r3 * u(4) * (u(3) - u(1)) + A * r1/r3 * u(4) * (u(3) - u(2))
  Divide : Product  Inputs=*/  OutScaling=2^-10
  Enthalpy_inlet : Fcn  Expr=u(1) * u(2)
  Enthalpy_outlet : Fcn  Expr=Ac * u(1) / dVc * u(2)
  Exchange_Cell : Fcn  Expr=u(1) * (-1.2290e4 + 35.12 * u(2))
  "JsO2, Tair" : Selector  Elements=[4 18]  InputPortWidth=28
  Mux1 : Mux  Inputs=2
  Mux2 : Mux  Inputs=2
  Mux3 : Mux  Inputs=2
  "NN2, NO2, Tair" : Selector  Elements=[25 26 18]  InputPortWidth=28
  Nj * Hj : Fcn  Expr="u(1)  *  (-1.0590e4 + 31.40 * u(3)) +  u(2) * (-1.2290e4 + 35.12 * u(3))"
  Pin Tin Uin : Selector  Elements=[10 11 12]  InputPortWidth=16
  Product : Product
  Sum : Sum  Inputs=+----
  Tair : Selector  Elements=[18]  InputPortWidth=28
  "Tcell, Ttube, Tair" : Selector  Elements=[15 16 18]  InputPortWidth=28
  Uair : Selector  Elements=[28]  InputPortWidth=28
  Xi * Hi : Fcn  Expr="(1-u(1)) * (-1.0590e4 + 31.40 * u(2))  + u(1) * (-1.2290e4 + 35.12 * u(2))"
  dotNin : Fcn  Expr=Ac * u(1) / R / u(2) * u(3)
  in{,1..3} (4 alike) : Display
  inlet fraction : Selector  Elements=[13 11]  InputPortWidth=16
  dot x18 : Outport
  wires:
  air (Ni*Cvi)/1 -> Divide/2
  Exchange_Cell/1 -> Sum/3, in3/1
  hc/1 -> Mux3/2
  "JsO2, Tair"/1 -> Exchange_Cell/1
  dotNin/1 -> Mux1/2
  Xi * Hi/1 -> Mux1/1
  Pin Tin Uin/1 -> dotNin/1
  x/1 -> "NN2, NO2, Tair"/1, "JsO2, Tair"/1, "Tcell, Ttube, Tair"/1, Tair/1, Uair/1
  inlet fraction/1 -> Xi * Hi/1
  Mux1/1 -> Enthalpy_inlet/1
  Mux3/1 -> Convection/1
  "Tcell, Ttube, Tair"/1 -> Mux3/1
  u/1 -> Pin Tin Uin/1, inlet fraction/1
  Enthalpy_inlet/1 -> Sum/1, in/1
  Enthalpy_outlet/1 -> Sum/2, in1/1
  Convection/1 -> Sum/4, in2/1
  Sum/1 -> Divide/1
  Divide/1 -> dot x18/1
  Mux2/1 -> Enthalpy_outlet/1
  "NN2, NO2, Tair"/1 -> Nj * Hj/1
  Nj * Hj/1 -> Mux2/1
  Uair/1 -> Mux2/2
  air d(Ni*Cvi)/1 -> Product/2
  Tair/1 -> Product/1
  Product/1 -> Sum/5

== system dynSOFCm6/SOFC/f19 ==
  note: [W]
  note: [W]
  note: [W]
  note: u14-16
  note: x19
  x : Inport  Port=1  LatchInput=off
  u : Inport  Port=2  LatchInput=off
  ht : Inport  Port=3  LatchInput=off
  inj (Ni*Cvi) : Inport  Port=4  LatchInput=off
  Convection_fuel : Fcn  Expr=u(3) * (u(2) - u(1)) * A * r0 / r3
  Divide : Product  Inputs=*/  OutScaling=2^-10
  Enthalpy : Fcn  Expr=-1.229e4 + 35.12*u(2)
  Enthalpy1 : Fcn  Expr=-1.229e4 + 35.12*u(1)
  Enthalpy_inlet : Fcn  Expr=u(1) * u(2)
  Enthalpy_outlet : Fcn  Expr=u(1) * u(2)
  Mux1 : Mux  Inputs=2
  Mux2 : Mux  Inputs=2
  Mux3 : Mux  Inputs=3
  Pinj Tinj Uinj : Selector  Elements=[14 15 16]  InputPortWidth=16
  Sum : Sum  Inputs=+--
  Tinj : Selector  Elements=[19]  InputPortWidth=28
  Ttube : Selector  Elements=[16]  InputPortWidth=28
  dotNin : Fcn  Expr=At * u(1) /(R * u(2)) * u(3)
  in : Display
  in1 : Display
  in2 : Display
  dot x19 : Outport
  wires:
  Divide/1 -> dot x19/1
  Sum/1 -> Divide/1
  Convection_fuel/1 -> in2/1, Sum/3
  Enthalpy_outlet/1 -> in1/1, Sum/2
  Enthalpy_inlet/1 -> in/1, Sum/1
  u/1 -> Pinj Tinj Uinj/1
  Mux3/1 -> Convection_fuel/1
  x/1 -> Tinj/1, Ttube/1
  Pinj Tinj Uinj/1 -> dotNin/1, Enthalpy/1
  Tinj/1 -> Enthalpy1/1, Mux3/2
  Ttube/1 -> Mux3/1
  ht/1 -> Mux3/3
  inj (Ni*Cvi)/1 -> Divide/2
  Enthalpy/1 -> Mux1/1
  dotNin/1 -> Mux1/2, Mux2/1
  Mux1/1 -> Enthalpy_inlet/1
  Mux2/1 -> Enthalpy_outlet/1
  Enthalpy1/1 -> Mux2/2

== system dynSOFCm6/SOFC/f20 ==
  note: u2-5
  note: [mol/s]
  note: [mol/s]
  note: [mol/m^2.s]
  note: x20,27
  note: x20,21,17
  x : Inport  Port=1  LatchInput=off
  u : Inport  Port=2  LatchInput=off
  Gain : Gain  Gain=A
  Gain1 : Gain  Gain=A
  "NCH4, NH2O, Tfuel" : Selector  Elements=[20 21 17]  InputPortWidth=28
  "NCH4, Ufuel" : Selector  Elements=[20 27]  InputPortWidth=28
  "NH2O, NCO, NH2, NCO2, Tfuel" : Selector  Elements="[21  23  22 24 17]"  InputPortWidth=28
  Nin : Fcn  Expr=Aa * u(1) /(R * u(2)) * u(3) * u(4)
  Nout : Fcn  Expr=Aa * u(1) / dVa * u(2)
  Pfuel Tfuel Ufuel XCH4 : Selector  Elements=[2 3 4 5]  InputPortWidth=16
  Reforming : Fcn  Expr=8542 * (u(1) * R * u(3) / dVa )^(0.85) * (u(2) * R * u(3) / dVa )^(-0.35) * exp( -95e3 /(8.314*u(3)) )
  Shifting : Fcn  Expr="100 * ( exp( 4276/u(5) - 3.961) * ( u(1) * R * u(5) / dVa ) * ( u(2) * R * u(5) / dVa ) -  (u(3) * R * u(5) / dVa ) * (u(4) * R * u(5) / dVa )  )"
  Sum : Sum  Inputs=+--
  r1 : Display
  r2 : Display
  dot x20 : Outport
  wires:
  Nin/1 -> Sum/1
  Pfuel Tfuel Ufuel XCH4/1 -> Nin/1
  x/1 -> "NCH4, Ufuel"/1, "NCH4, NH2O, Tfuel"/1, "NH2O, NCO, NH2, NCO2, Tfuel"/1
  u/1 -> Pfuel Tfuel Ufuel XCH4/1
  "NCH4, Ufuel"/1 -> Nout/1
  "NCH4, NH2O, Tfuel"/1 -> Reforming/1
  "NH2O, NCO, NH2, NCO2, Tfuel"/1 -> Shifting/1
  Reforming/1 -> Gain/1
  Sum/1 -> dot x20/1
  Shifting/1 -> Gain1/1
  Gain1/1 -> r2/1
  Nout/1 -> Sum/2
  Gain/1 -> Sum/3, r1/1

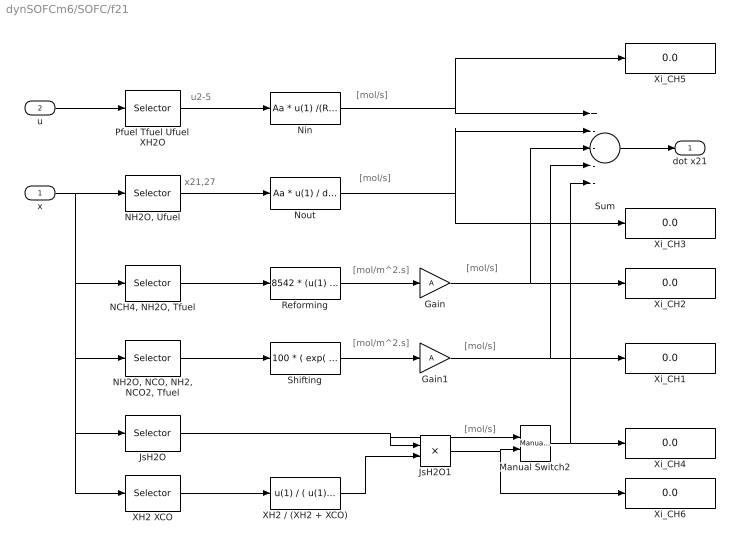
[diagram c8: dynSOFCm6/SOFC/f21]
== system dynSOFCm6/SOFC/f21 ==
  note: [mol/m^2.s]
  note: [mol/s]
  note: [mol/s]
  note: u2-5
  note: [mol/m^2.s]
  note: [mol/s]
  note: [mol/s]
  note: [mol/s]
  note: x21,27
  x : Inport  Port=1  LatchInput=off
  u : Inport  Port=2  LatchInput=off
  Gain : Gain  Gain=A
  Gain1 : Gain  Gain=A
  JsH2O : Selector  Elements=[6]  InputPortWidth=28
  JsH2O1 : Product  Inputs=**  OutScaling=2^-10
  Manual Switch2 : simulink/Signal Routing/Manual Switch  sw=1  action=0
  "NCH4, NH2O, Tfuel" : Selector  Elements=[20 21 17]  InputPortWidth=28
  "NH2O, NCO, NH2, NCO2, Tfuel" : Selector  Elements="[21  23  22 24 17]"  InputPortWidth=28
  "NH2O, Ufuel" : Selector  Elements=[21 27]  InputPortWidth=28
  Nin : Fcn  Expr=Aa * u(1) /(R * u(2)) * u(3) * u(4)
  Nout : Fcn  Expr=Aa * u(1) / dVa * u(2)
  Pfuel Tfuel Ufuel XH2O : Selector  Elements=[2 3 4 6]  InputPortWidth=16
  Reforming : Fcn  Expr=8542 * (u(1) * R * u(3) / dVa )^(0.85) * (u(2) * R * u(3) / dVa )^(-0.35) * exp( -95e3 /(8.314*u(3)) )
  Shifting : Fcn  Expr="100 * ( exp( 4276/u(5) - 3.961) * ( u(1) * R * u(5) / dVa ) * ( u(2) * R * u(5) / dVa ) -  (u(3) * R * u(5) / dVa ) * (u(4) * R * u(5) / dVa )  )"
  Sum : Sum  Inputs=+----
  XH2 / (XH2 + XCO) : Fcn  Expr=u(1) / ( u(1) + u(2))
  XH2 XCO : Selector  Elements=[22 23]  InputPortWidth=28
  Xi_CH{1..6} (6 alike) : Display
  dot x21 : Outport
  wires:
  Sum/1 -> dot x21/1
  Gain/1 -> Xi_CH2/1, Sum/3
  Reforming/1 -> Gain/1
  Nout/1 -> Xi_CH3/1, Sum/2
  "NH2O, NCO, NH2, NCO2, Tfuel"/1 -> Shifting/1
  "NCH4, NH2O, Tfuel"/1 -> Reforming/1
  "NH2O, Ufuel"/1 -> Nout/1
  u/1 -> Pfuel Tfuel Ufuel XH2O/1
  x/1 -> "NH2O, NCO, NH2, NCO2, Tfuel"/1, JsH2O/1, XH2 XCO/1, "NCH4, NH2O, Tfuel"/1, "NH2O, Ufuel"/1
  Pfuel Tfuel Ufuel XH2O/1 -> Nin/1
  Nin/1 -> Xi_CH5/1, Sum/1
  Shifting/1 -> Gain1/1
  Gain1/1 -> Xi_CH1/1, Sum/4
  JsH2O/1 -> Manual Switch2/1, JsH2O1/1
  XH2 / (XH2 + XCO)/1 -> JsH2O1/2
  XH2 XCO/1 -> XH2 / (XH2 + XCO)/1
  Manual Switch2/1 -> Xi_CH4/1, Sum/5
  JsH2O1/1 -> Manual Switch2/2, Xi_CH6/1

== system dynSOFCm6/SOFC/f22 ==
  note: [mol/s]
  note: [mol/s]
  note: [mol/s]
  note: [mol/m^2.s]
  note: u2-5
  note: [mol/s]
  note: [mol/s]
  note: [mol/m^2.s]
  x : Inport  Port=1  LatchInput=off
  u : Inport  Port=2  LatchInput=off
  Divide2 : Product  Inputs=**  OutScaling=2^-10
  Gain : Gain  Gain=3*A
  Gain1 : Gain  Gain=A
  JsH2 : Selector  Elements=[2]  InputPortWidth=28
  Manual Switch2 : simulink/Signal Routing/Manual Switch  sw=1  action=0
  "NCH4, NH2O, Tfuel" : Selector  Elements=[20 21 17]  InputPortWidth=28
  "NH2, Ufuel" : Selector  Elements=[22 27]  InputPortWidth=28
  "NH2O, NCO, NH2, NCO2, Tfuel" : Selector  Elements="[21  23  22 24 17]"  InputPortWidth=28
  Nin : Fcn  Expr=Aa * u(1) /(R * u(2)) * u(3) * u(4)
  Nout : Fcn  Expr=Aa * u(1) / dVa * u(2)
  Pfuel Tfuel Ufuel XH2 : Selector  Elements=[2 3 4 7]  InputPortWidth=16
  Reforming : Fcn  Expr=8542 * (u(1) * R * u(3) / dVa )^(0.85) * (u(2) * R * u(3) / dVa )^(-0.35) * exp( -95e3 /(8.314*u(3)) )
  Shifting : Fcn  Expr="100 * ( exp( 4276/u(5) - 3.961) * ( u(1) * R * u(5) / dVa ) * ( u(2) * R * u(5) / dVa ) -  (u(3) * R * u(5) / dVa ) * (u(4) * R * u(5) / dVa )  )"
  Sum : Sum  Inputs=+-++-
  XH2 / (XH2 + XCO) : Fcn  Expr=u(1) / ( u(1) + u(2))
  XH2 XCO : Selector  Elements=[22 23]  InputPortWidth=28
  Xi_O{1..5} (5 alike) : Display
  dot x22 : Outport
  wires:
  Shifting/1 -> Gain1/1
  Nin/1 -> Xi_O5/1, Sum/1
  Pfuel Tfuel Ufuel XH2/1 -> Nin/1
  x/1 -> "NH2, Ufuel"/1, "NH2O, NCO, NH2, NCO2, Tfuel"/1, JsH2/1, XH2 XCO/1, "NCH4, NH2O, Tfuel"/1
  u/1 -> Pfuel Tfuel Ufuel XH2/1
  "NH2, Ufuel"/1 -> Nout/1
  "NCH4, NH2O, Tfuel"/1 -> Reforming/1
  "NH2O, NCO, NH2, NCO2, Tfuel"/1 -> Shifting/1
  Nout/1 -> Xi_O4/1, Sum/2
  Reforming/1 -> Gain/1
  Gain/1 -> Xi_O3/1, Sum/3
  Sum/1 -> dot x22/1
  Gain1/1 -> Xi_O1/1, Sum/4
  XH2 / (XH2 + XCO)/1 -> Divide2/2
  JsH2/1 -> Divide2/1, Manual Switch2/1
  XH2 XCO/1 -> XH2 / (XH2 + XCO)/1
  Manual Switch2/1 -> Xi_O2/1, Sum/5
  Divide2/1 -> Manual Switch2/2

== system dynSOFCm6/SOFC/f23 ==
  note: [mol/m^2.s]
  note: [mol/s]
  note: [mol/s]
  note: [mol/m^2.s]
  note: [mol/s]
  note: [mol/s]
  note: [mol/s]
  x : Inport  Port=1  LatchInput=off
  u : Inport  Port=2  LatchInput=off
  Constant2 : Constant  Value=0
  Gain : Gain  Gain=A
  Gain1 : Gain  Gain=A
  JsCO : Product  Inputs=**  OutScaling=2^-10
  JsH2 : Selector  Elements=[3]  InputPortWidth=28
  Manual Switch2 : simulink/Signal Routing/Manual Switch  sw=1  action=0
  "NCH4, NH2O, Tfuel" : Selector  Elements=[20 21 17]  InputPortWidth=28
  "NCO, Ufuel" : Selector  Elements=[23 27]  InputPortWidth=28
  "NH2O, NCO, NH2, NCO2, Tfuel" : Selector  Elements="[21  23  22 24 17]"  InputPortWidth=28
  Nin : Fcn  Expr=Aa * u(1) /(R * u(2)) * u(3) * u(4)
  Nout : Fcn  Expr=Aa * u(1) / dVa * u(2)
  Pfuel Tfuel Ufuel XCO : Selector  Elements=[2 3 4 8]  InputPortWidth=16
  Reforming : Fcn  Expr=8542 * (u(1) * R * u(3) / dVa )^(0.85) * (u(2) * R * u(3) / dVa )^(-0.35) * exp( -95e3 /(8.314*u(3)) )
  Shifting : Fcn  Expr="100 * ( exp( 4276/u(5) - 3.961) * ( u(1) * R * u(5) / dVa ) * ( u(2) * R * u(5) / dVa ) -  (u(3) * R * u(5) / dVa ) * (u(4) * R * u(5) / dVa )  )"
  Sum : Sum  Inputs=+-+--
  XCO / (XH2 + XCO) : Fcn  Expr=u(2) / ( u(1) + u(2))
  XH2 XCO : Selector  Elements=[22 23]  InputPortWidth=28
  dot x23 : Outport
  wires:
  Sum/1 -> dot x23/1
  Reforming/1 -> Gain/1
  "NH2O, NCO, NH2, NCO2, Tfuel"/1 -> Shifting/1
  "NCH4, NH2O, Tfuel"/1 -> Reforming/1
  "NCO, Ufuel"/1 -> Nout/1
  u/1 -> Pfuel Tfuel Ufuel XCO/1
  x/1 -> "NCH4, NH2O, Tfuel"/1, "NH2O, NCO, NH2, NCO2, Tfuel"/1, JsH2/1, XH2 XCO/1, "NCO, Ufuel"/1
  Pfuel Tfuel Ufuel XCO/1 -> Nin/1
  Nin/1 -> Sum/1
  Shifting/1 -> Gain1/1
  Nout/1 -> Sum/2
  Gain1/1 -> Sum/4
  Gain/1 -> Sum/3
  JsH2/1 -> JsCO/1
  XH2 XCO/1 -> XCO / (XH2 + XCO)/1
  XCO / (XH2 + XCO)/1 -> JsCO/2
  Manual Switch2/1 -> Sum/5
  JsCO/1 -> Manual Switch2/2
  Constant2/1 -> Manual Switch2/1

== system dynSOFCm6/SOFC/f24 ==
  note: [mol/s]
  note: [mol/s]
  note: [mol/m^2.s]
  note: [mol/s]
  note: [mol/s]
  note: [mol/m^2.s]
  note: [mol/s]
  x : Inport  Port=1  LatchInput=off
  u : Inport  Port=2  LatchInput=off
  Constant2 : Constant  Value=0
  Gain : Gain  Gain=A
  Gain1 : Gain  Gain=A
  JsCO2 : Product  Inputs=**  OutScaling=2^-10
  JsH2 : Selector  Elements=[3]  InputPortWidth=28
  Manual Switch2 : simulink/Signal Routing/Manual Switch  sw=1  action=0
  "NCH4, NH2O, Tfuel1" : Selector  Elements=[20 21 17]  InputPortWidth=28
  "NCO2, Ufuel" : Selector  Elements=[24 27]  InputPortWidth=28
  "NH2O, NCO, NH2, NCO2, Tfuel1" : Selector  Elements="[21  23  22 24 17]"  InputPortWidth=28
  Nin : Fcn  Expr=Aa * u(1) /(R * u(2)) * u(3) * u(4)
  Nout : Fcn  Expr=Aa * u(1) / dVa * u(2)
  Pfuel Tfuel Ufuel XCO2 : Selector  Elements=[2 3 4 9]  InputPortWidth=16
  Reforming : Fcn  Expr=8542 * (u(1) * R * u(3) / dVa )^(0.85) * (u(2) * R * u(3) / dVa )^(-0.35) * exp( -95e3 /(8.314*u(3)) )
  Shifting : Fcn  Expr="100 * ( exp( 4276/u(5) - 3.961) * ( u(1) * R * u(5) / dVa ) * ( u(2) * R * u(5) / dVa ) -  (u(3) * R * u(5) / dVa ) * (u(4) * R * u(5) / dVa )  )"
  Sum : Sum  Inputs=+-++
  XCO / (XH2 + XCO) : Fcn  Expr=u(2) / ( u(1) + u(2))
  XH2 XCO : Selector  Elements=[22 23]  InputPortWidth=28
  dot x24 : Outport
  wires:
  Shifting/1 -> Gain1/1
  Nin/1 -> Sum/1
  Pfuel Tfuel Ufuel XCO2/1 -> Nin/1
  x/1 -> "NCO2, Ufuel"/1, "NCH4, NH2O, Tfuel1"/1, "NH2O, NCO, NH2, NCO2, Tfuel1"/1, JsH2/1, XH2 XCO/1
  u/1 -> Pfuel Tfuel Ufuel XCO2/1
  "NCO2, Ufuel"/1 -> Nout/1
  "NCH4, NH2O, Tfuel1"/1 -> Reforming/1
  "NH2O, NCO, NH2, NCO2, Tfuel1"/1 -> Shifting/1
  Reforming/1 -> Gain/1
  Sum/1 -> dot x24/1
  Nout/1 -> Sum/2
  Gain1/1 -> Sum/3
  JsH2/1 -> JsCO2/1
  XH2 XCO/1 -> XCO / (XH2 + XCO)/1
  XCO / (XH2 + XCO)/1 -> JsCO2/2
  Manual Switch2/1 -> Sum/4
  JsCO2/1 -> Manual Switch2/2
  Constant2/1 -> Manual Switch2/1

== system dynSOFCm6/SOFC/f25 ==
  note: [mol/s]
  note: [mol/s]
  x : Inport  Port=1  LatchInput=off
  u : Inport  Port=2  LatchInput=off
  "NN2, Uair" : Selector  Elements=[25 28]  InputPortWidth=28
  Nin : Fcn  Expr=Ac * u(1) /(R * u(2)) * u(3) * (1 - u(4))
  Nout : Fcn  Expr=Ac * u(1) / dVc * u(2)
  Pair Tair Uair XO2 : Selector  Elements=[10 11 12 13]  InputPortWidth=16
  Sum : Sum  Inputs=+-
  Xi_O1 : Display
  Xi_O4 : Display
  dot x25 : Outport
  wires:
  Nin/1 -> Sum/1, Xi_O4/1
  Pair Tair Uair XO2/1 -> Nin/1
  x/1 -> "NN2, Uair"/1
  u/1 -> Pair Tair Uair XO2/1
  "NN2, Uair"/1 -> Nout/1
  Nout/1 -> Sum/2, Xi_O1/1
  Sum/1 -> dot x25/1

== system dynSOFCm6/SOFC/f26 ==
  note: [mol/s]
  note: [mol/s]
  note: [mol/s]
  x : Inport  Port=1  LatchInput=off
  u : Inport  Port=2  LatchInput=off
  JsO2 : Selector  Elements=[4]  InputPortWidth=28
  "NO2, Uair" : Selector  Elements=[26 28]  InputPortWidth=28
  Nin : Fcn  Expr=Ac * u(1) /(R * u(2)) * u(3) * u(4)
  Nout : Fcn  Expr=Ac * u(1) / dVc * u(2)
  Pair Tair Uair XO2 : Selector  Elements=[10 11 12 13]  InputPortWidth=16
  Sum : Sum  Inputs=+--
  Xi_O1 : Display
  Xi_O2 : Display
  Xi_O4 : Display
  dot x26 : Outport
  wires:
  JsO2/1 -> Sum/3, Xi_O2/1
  Nout/1 -> Sum/2, Xi_O1/1
  "NO2, Uair"/1 -> Nout/1
  u/1 -> Pair Tair Uair XO2/1
  x/1 -> "NO2, Uair"/1, JsO2/1
  Pair Tair Uair XO2/1 -> Nin/1
  Nin/1 -> Sum/1, Xi_O4/1
  Sum/1 -> dot x26/1

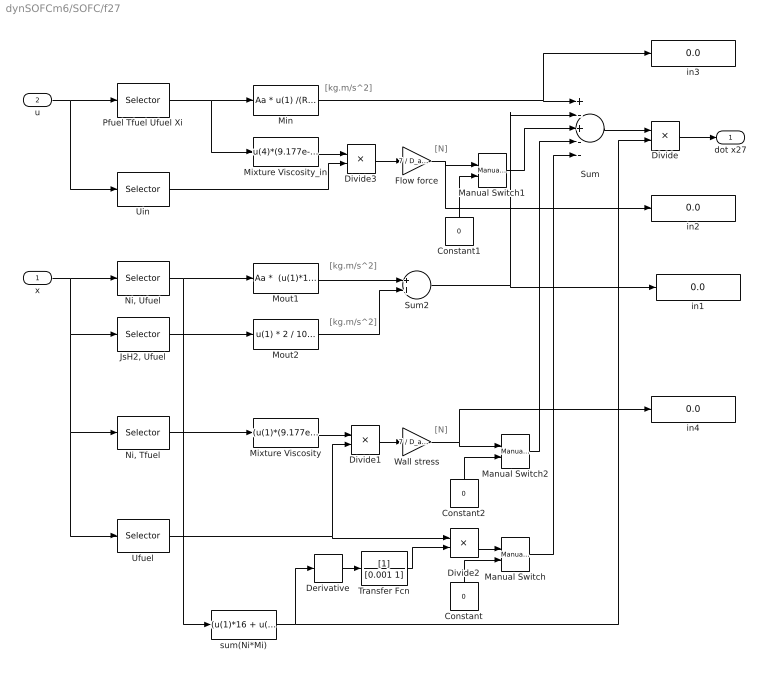
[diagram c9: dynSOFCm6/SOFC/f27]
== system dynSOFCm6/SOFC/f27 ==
  note: [kg.m/s^2]
  note: [kg.m/s^2]
  note: [N]
  note: [N]
  note: [kg.m/s^2]
  x : Inport  Port=1  LatchInput=off
  u : Inport  Port=2  LatchInput=off
  Constant : Constant  Orientation=up  Value=0
  Constant1 : Constant  Orientation=up  Value=0
  Constant2 : Constant  Orientation=up  Value=0
  Derivative : Derivative
  Divide : Product  Inputs=*/  OutScaling=2^-10
  Divide1 : Product  Inputs=**  OutScaling=2^-10
  Divide2 : Product  Inputs=**  OutScaling=2^-10
  Divide3 : Product  Inputs=**  OutScaling=2^-10
  Flow force : Gain  Gain=7 / D_a * A *1.2
  "JsH2, Ufuel" : Selector  Elements=[2 27]  InputPortWidth=28
  Manual Switch : simulink/Signal Routing/Manual Switch  sw=1  action=0
  Manual Switch1 : simulink/Signal Routing/Manual Switch  sw=0  action=0
  Manual Switch2 : simulink/Signal Routing/Manual Switch  sw=0  action=0
  Min : Fcn  Expr=Aa * u(1) /(R * u(2)) * (u(4)*16 + u(5)*18 + u(6)*2 + u(7)*28 + u(8)*44)/1000 * u(3)^2
  Mixture Viscosity : Fcn  Expr="(u(1)*(9.177e-6 + 1.755e-8*u(6)) +  u(2)*(4.567e-6 + 2.209e-8*u(6)) + u(3)*(6.162e-6 + 1.145e-8*u(6)) + u(4)*(1.399e-5 + 2.582e-8*u(6)) + u(5)*(1.273e-5 + 2.822e-8*u(6)) ) / (u(1) +u(2) + u(3) + u(4) +u(5) )"
  Mixture Viscosity_in : Fcn  Expr="u(4)*(9.177e-6 + 1.755e-8*u(2)) +  u(5)*(4.567e-6 + 2.209e-8*u(2)) + u(6)*(6.162e-6 + 1.145e-8*u(2)) + u(7)*(1.399e-5 + 2.582e-8*u(2)) + u(8)*(1.273e-5 + 2.822e-8*u(2))"
  Mout1 : Fcn  Expr="Aa *  (u(1)*16 + u(2)*18 + u(3)*2 + u(4)*28 + u(5)*44)/1000 / dVa * u(6)^2"
  Mout2 : Fcn  Expr="u(1) * 2 / 1000  * u(2)"
  "Ni, Tfuel" : Selector  Elements=[20 21 22 23 24 17]  InputPortWidth=28
  "Ni, Ufuel" : Selector  Elements=[20 21 22 23 24 27]  InputPortWidth=28
  Pfuel Tfuel Ufuel Xi : Selector  Elements=[2 3 4 5 6 7 8 9]  InputPortWidth=16
  Sum : Sum  Inputs=+-+--
  Sum2 : Sum
  Transfer Fcn : TransferFcn  Denominator=[0.001 1]
  Ufuel : Selector  Elements=[27]  InputPortWidth=28
  Uin : Selector  Elements=[4]  InputPortWidth=16
  Wall stress : Gain  Gain=7 / D_a * A
  in{1..4} (4 alike) : Display
  sum(Ni*Mi) : Fcn  Expr=(u(1)*16 + u(2)*18 + u(3)*2 + u(4)*28 + u(5)*44)/1000
  dot x27 : Outport
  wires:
  "Ni, Tfuel"/1 -> Mixture Viscosity/1
  "Ni, Ufuel"/1 -> Mout1/1, sum(Ni*Mi)/1
  u/1 -> Pfuel Tfuel Ufuel Xi/1, Uin/1
  x/1 -> "Ni, Ufuel"/1, "Ni, Tfuel"/1, Ufuel/1, "JsH2, Ufuel"/1
  Pfuel Tfuel Ufuel Xi/1 -> Min/1, Mixture Viscosity_in/1
  Min/1 -> Sum/1, in3/1
  Divide3/1 -> Flow force/1
  sum(Ni*Mi)/1 -> Derivative/1, Divide/2
  Manual Switch/1 -> Sum/5
  Sum/1 -> Divide/1
  Mixture Viscosity/1 -> Divide1/1
  Divide1/1 -> Wall stress/1
  Manual Switch2/1 -> Sum/4
  Wall stress/1 -> Manual Switch2/1, in4/1
  Constant/1 -> Manual Switch/2
  Ufuel/1 -> Divide1/2, Divide2/1
  "JsH2, Ufuel"/1 -> Mout2/1
  Mout1/1 -> Sum2/1
  Mout2/1 -> Sum2/2
  Sum2/1 -> Sum/2, in1/1
  Manual Switch1/1 -> Sum/3
  Divide2/1 -> Manual Switch/1
  Mixture Viscosity_in/1 -> Divide3/1
  Uin/1 -> Divide3/2
  Flow force/1 -> Manual Switch1/1, in2/1
  Constant2/1 -> Manual Switch2/2
  Constant1/1 -> Manual Switch1/2
  Divide/1 -> dot x27/1
  Derivative/1 -> Transfer Fcn/1
  Transfer Fcn/1 -> Divide2/2

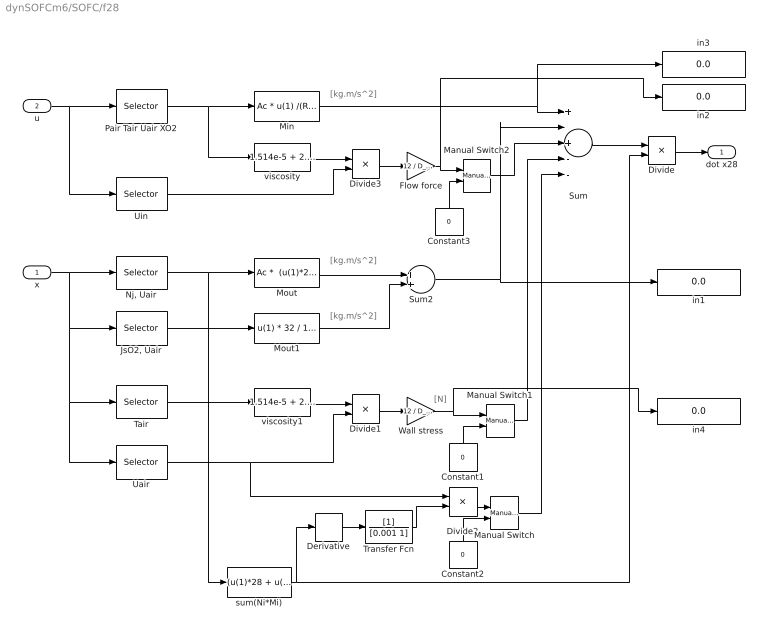
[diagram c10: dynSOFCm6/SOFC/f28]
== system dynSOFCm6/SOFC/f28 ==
  note: [N]
  note: [kg.m/s^2]
  note: [kg.m/s^2]
  note: [kg.m/s^2]
  x : Inport  Port=1  LatchInput=off
  u : Inport  Port=2  LatchInput=off
  Constant1 : Constant  Orientation=up  Value=0
  Constant2 : Constant  Orientation=up  Value=0
  Constant3 : Constant  Orientation=up  Value=0
  Derivative : Derivative
  Divide : Product  Inputs=*/  OutScaling=2^-10
  Divide1 : Product  Inputs=**  OutScaling=2^-10
  Divide2 : Product  Inputs=**  OutScaling=2^-10
  Divide3 : Product  Inputs=**  OutScaling=2^-10
  Flow force : Gain  Gain=12 / D_c * A * (r2 + r1) / r3
  "JsO2, Uair" : Selector  Elements=[4 28]  InputPortWidth=28
  Manual Switch : simulink/Signal Routing/Manual Switch  sw=1  action=0
  Manual Switch1 : simulink/Signal Routing/Manual Switch  sw=0  action=0
  Manual Switch2 : simulink/Signal Routing/Manual Switch  sw=0  action=0
  Min : Fcn  Expr=Ac * u(1) /(R * u(2)) * ( (1-u(4)) * 28 + u(4)*32 )/1000 * u(3)^2
  Mout : Fcn  Expr="Ac *  (u(1)*28 + u(2)*32 )/1000 / dVc * u(3)^2"
  Mout1 : Fcn  Expr="u(1) * 32 / 1000  * u(2)"
  "Nj, Uair" : Selector  Elements=[25 26 28]  InputPortWidth=28
  Pair Tair Uair XO2 : Selector  Elements=[10 11 12 13]  InputPortWidth=16
  Sum : Sum  Inputs=+-+--
  Sum2 : Sum
  Tair : Selector  Elements=[18]  InputPortWidth=28
  Transfer Fcn : TransferFcn  Denominator=[0.001 1]
  Uair : Selector  Elements=[28]  InputPortWidth=28
  Uin : Selector  Elements=[12]  InputPortWidth=16
  Wall stress : Gain  Gain=12 / D_c * A * (r2 + r1) / r3
  in{1..4} (4 alike) : Display
  sum(Ni*Mi) : Fcn  Expr=(u(1)*28 + u(2)*32 )/1000
  viscosity : Fcn  Expr=1.514e-5 + 2.793e-8*u(2)
  viscosity1 : Fcn  Expr=1.514e-5 + 2.793e-8*u(1)
  dot x28 : Outport
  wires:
  Sum/1 -> Divide/1
  sum(Ni*Mi)/1 -> Divide/2, Derivative/1
  Uin/1 -> Divide3/2
  Min/1 -> Sum/1, in3/1
  Pair Tair Uair XO2/1 -> Min/1, viscosity/1
  x/1 -> "Nj, Uair"/1, "JsO2, Uair"/1, Uair/1, Tair/1
  u/1 -> Uin/1, Pair Tair Uair XO2/1
  "Nj, Uair"/1 -> Mout/1, sum(Ni*Mi)/1
  Uair/1 -> Divide1/2, Divide2/1
  Manual Switch/1 -> Sum/5
  Divide3/1 -> Flow force/1
  viscosity/1 -> Divide3/1
  "JsO2, Uair"/1 -> Mout1/1
  Mout/1 -> Sum2/1
  Divide1/1 -> Wall stress/1
  Tair/1 -> viscosity1/1
  viscosity1/1 -> Divide1/1
  Sum2/1 -> Sum/2, in1/1
  Manual Switch1/1 -> Sum/4
  Divide2/1 -> Manual Switch/1
  Wall stress/1 -> Manual Switch1/1, in4/1
  Constant1/1 -> Manual Switch1/2
  Constant2/1 -> Manual Switch/2
  Flow force/1 -> Manual Switch2/1, in2/1
  Constant3/1 -> Manual Switch2/2
  Manual Switch2/1 -> Sum/3
  Mout1/1 -> Sum2/2
  Divide/1 -> dot x28/1
  Derivative/1 -> Transfer Fcn/1
  Transfer Fcn/1 -> Divide2/2
